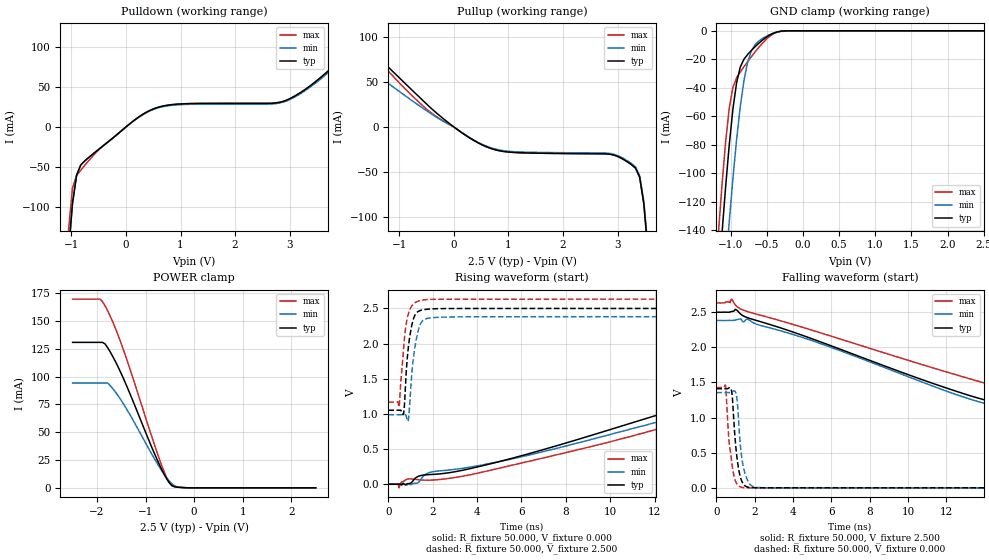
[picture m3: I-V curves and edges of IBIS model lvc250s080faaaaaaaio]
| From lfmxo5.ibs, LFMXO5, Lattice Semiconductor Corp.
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[Model] lvc250s080faaaaaaaio
Model_type I/O
Polarity   Non-Inverting
Enable   Active-Low
Vinl =  0.700V
Vinh =  1.700V
Vmeas =  1.250V
Cref =  0.0F
Rref =  1.000M
Vref =  0.0V
C_comp   5.000pF   4.000pF   5.500pF
[Temperature Range]   25.000   0.125k   -40.000
[Voltage Range]   2.500V   2.380V   2.630V
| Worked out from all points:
|   slope of the pulldown table from 0 to 0.375 V, typ, clamps not added: 20.3 ohm
|   slope of the pullup table from 0 to 0.375 V, typ, clamps not added: 24.5 ohm
|   GND clamp passes 1 mA (typ) near -0.37 V on its own axis
|   POWER clamp passes 1 mA (typ) near -0.40 V on its own axis
|   rising waveform, R_fixture 50.000, V_fixture 0.000: 20-80 % time 9.28ns typ, 10.6ns min, 10ns max; typ from 0 V to 1.41 V
|   rising waveform, R_fixture 50.000, V_fixture 2.500: 20-80 % time 263ps typ, 298ps min, 275ps max; typ from 1.05 V to 2.5 V
|   falling waveform, R_fixture 50.000, V_fixture 2.500: 20-80 % time 8.81ns typ, 8.29ns min, 10.6ns max; typ from 2.5 V to 1.05 V
|   falling waveform, R_fixture 50.000, V_fixture 0.000: 20-80 % time 281ps typ, 298ps min, 288ps max; typ from 1.41 V to 0 V
[GND_clamp]
|Voltage   I(typ)   I(min)   I(max)
-2.5V     -1.233A    -1.246A    -1.23A
-1.174V   -179.1mA   -235.9mA   -144.4mA
-1.123V   -143.6mA   -200.7mA   -109.5mA
-1.072V   -110.2mA   -166.6mA   -78.57mA
-1.021V   -80.08mA   -134.1mA   -54.34mA
-970mV    -54.89mA   -103.7mA   -39.63mA
-919mV    -36.41mA   -76.3mA    -32.99mA
-817mV    -19.89mA   -34.81mA   -25.2mA
-715mV    -13.78mA   -14.11mA   -18.16mA
-511mV    -4.596mA   -3.904mA   -6.102mA
-256mV    -63.21uA   -177.9uA   -38.32uA
2.5V      -23.56nA   0A         -150.9nA
[POWER_clamp]
|Voltage   I(typ)   I(min)   I(max)
-2.5V     130.9mA    94.41mA    169.8mA
-1.937V   130.9mA    94.41mA    169.8mA
-1.835V   129.6mA    94.41mA    163.9mA
-1.733V   122.8mA    92.29mA    155mA
-1.478V   100.7mA    77.18mA    127mA
-866mV    35.87mA    29.9mA     45.33mA
-662mV    16.03mA    15.02mA    19.46mA
-560mV    7.73mA     8.668mA    8.662mA
-458mV    2.143mA    3.687mA    1.896mA
-356mV    647.1uA    1.015mA    754.8uA
-101mV    23.95uA    66.65uA    14.28uA
2.5V      0A         0A         0A
[Pulldown]
|Voltage   I(typ)   I(min)   I(max)
-2.5V     -2.07A     -2.07A     -2.62A
-1.056V   -159.5mA   -159.5mA   -132.1mA
-980mV    -96.2mA    -96.2mA    -76.81mA
-904mV    -60.38mA   -60.38mA   -61.04mA
-828mV    -47.63mA   -47.63mA   -54.22mA
-448mV    -25.25mA   -25.25mA   -25.53mA
312mV     15.95mA    15.47mA    15.95mA
920mV     28.42mA    27.56mA    28.42mA
2.896V    32.3mA     31.33mA    32.3mA
3.428V    54.23mA    52.6mA     54.23mA
4.644V    124.9mA    121.2mA    124.9mA
5V        134mA      130mA      134mA
[Pullup]
|Voltage   I(typ)   I(min)   I(max)
-2.5V     105.7mA    79.6mA     120.1mA
-1.992V   103.8mA    77.3mA     110.7mA
-1.536V   85mA       62.39mA    83.9mA
-472mV    23.75mA    16.9mA     18.26mA
592mV     -21.87mA   -21.22mA   -21.87mA
1.124V    -28.36mA   -27.51mA   -28.36mA
2.796V    -29.88mA   -28.99mA   -29.88mA
3.1V      -35.75mA   -34.68mA   -35.75mA
3.328V    -45.66mA   -44.29mA   -45.66mA
3.404V    -55.72mA   -54.05mA   -55.72mA
3.556V    -138.2mA   -134.1mA   -138.2mA
5V        -1.766A    -1.713A    -1.766A
[Ramp]
| variable   typ   min   max
dV/dt_r   0.847/9.273n   0.813/10.559n   0.857/10.016n
dV/dt_f   0.868/8.811n   0.837/8.301n   0.878/10.585n
R_load = 50.000
[Rising Waveform]
R_fixture = 50.000
V_fixture = 0.000
V_fixture_min = 0.000
V_fixture_max = 0.000
|  time   V(typ)   V(min)   V(max)
0s        64.19uV    -272.3uV   349.5uV
436ps     151.5uV    -457.7uV   2.678mV
479ps     187.8uV    -278.7uV   -51.51mV
874ps     8.061mV    -1.916mV   74.2mV
1.334ns   110.4mV    21.91mV    65.41mV
1.914ns   138.3mV    172mV      58.59mV
4.194ns   259.4mV    271.8mV    169.3mV
11.03ns   877.9mV    793.8mV    688.9mV
14.95ns   1.218V     1.099V     1.063V
20ns      1.411V     1.355V     1.429V
[Rising Waveform]
R_fixture = 50.000
V_fixture = 2.500
V_fixture_min = 2.380
V_fixture_max = 2.630
|  time   V(typ)   V(min)   V(max)
0s        1.052V     987.3mV    1.168V
483ps     1.052V     987.1mV    1.101V
688ps     1.007V     987.6mV    1.935V
777ps     1.435V     984.6mV    2.221V
887ps     1.908V     899.9mV    2.408V
1.139ns   2.36V      1.82V      2.565V
1.257ns   2.433V     2.059V     2.591V
1.447ns   2.471V     2.278V     2.613V
2.567ns   2.498V     2.377V     2.631V
20ns      2.5V       2.383V     2.632V
[Falling Waveform]
R_fixture = 50.000
V_fixture = 2.500
V_fixture_min = 2.380
V_fixture_max = 2.630
|  time   V(typ)   V(min)   V(max)
0s        2.5V       2.383V     2.632V
721ps     2.503V     2.383V     2.635V
800ps     2.509V     2.383V     2.686V
998ps     2.54V      2.39V      2.603V
1.274ns   2.472V     2.403V     2.546V
1.414ns   2.447V     2.362V     2.529V
1.644ns   2.42V      2.4V       2.508V
14.21ns   1.236V     1.186V     1.476V
16.77ns   1.107V     1.058V     1.302V
20ns      1.052V     987.3mV    1.168V
[Falling Waveform]
R_fixture = 50.000
V_fixture = 0.000
V_fixture_min = 0.000
V_fixture_max = 0.000
|  time   V(typ)   V(min)   V(max)
0s        1.411V     1.355V     1.429V
486ps     1.411V     1.355V     1.449V
657ps     1.421V     1.355V     685.4mV
778ps     1.4V       1.359V     428.4mV
838ps     1.285V     1.367V     297.2mV
1.058ns   482.1mV    1.305V     63.92mV
1.308ns   110.5mV    473.9mV    9.185mV
1.644ns   10.41mV    100.8mV    404.4uV
2.104ns   775.5uV    6.884mV    -241.6uV
20ns      64.19uV    -272.3uV   349.5uV
